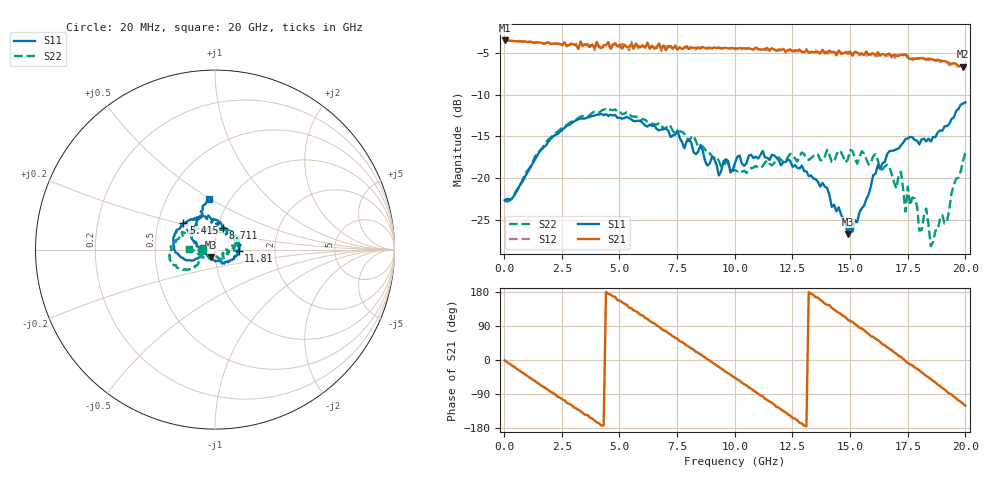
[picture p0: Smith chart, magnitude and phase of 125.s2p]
!Agilent Technologies,N5230A,US43500223,A.07.50.48
!Agilent N5230A: A.07.50.48
!Date: Tuesday, September 15, 2015 20:15:57
!Correction: S11(Full 2 Port(1,2))
!S21(Full 2 Port(1,2))
!S12(Full 2 Port(1,2))
!S22(Full 2 Port(1,2))
!S2P File: Measurements: S11, S21, S12, S22:
# Hz S  RI  R 50
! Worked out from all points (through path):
!   201 points, 20 MHz to 20 GHz, reference 50 ohm
!   highest |S21| = -3.50 dB at 20 MHz (marker M1); lowest = -6.6 dB at 19.9 GHz (marker M2)
!   group delay of S21, straight-line fit = 116 ps
!   lowest |S11| = -26.7 dB at 14.91 GHz (marker M3), VSWR 1.10, Z = 47.8 - j3.93 ohm
!   |S11| at or under -10 dB: start of sweep to end of sweep
!   |S22| runs from -28.2 to -11.7 dB; largest |S21 - S12| = 0.048
!   S11 on the Smith chart (normalised r, x): 20 MHz: 0.86, +0.00; 5.415 GHz: 0.67, +0.21; 8.711 GHz: 1.06, +0.26; 11.81 GHz: 1.31, -0.02; 20 GHz: 0.80, +0.49
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2e7  -0.0736 0.000765  0.668 -0.0104  0.668 -0.0107  -0.073 -0.000204
1.9181e9  -0.1538 -0.0604  0.119 -0.6413  0.1163 -0.6372  -0.1336 -0.1056
3.4166e9  -0.2271 0.0105  -0.4797 -0.3981  -0.4777 -0.3725  -0.214 -0.0977
4.5155e9  -0.2157 0.0958  -0.648 0.0598  -0.6482 0.0751  -0.2499 -0.0403
5.4146e9  -0.1758 0.147  -0.4542 0.4088  -0.45 0.3706  -0.2454 0.0158
6.7133e9  -0.0794 0.1765  0.0244 0.6407  0.0347 0.6339  -0.197 0.0809
8.7113e9  0.0435 0.119  0.5966 0.0685  0.5909 0.0716  -0.0951 0.1145
1.001e10  0.0965 0.0764  0.4062 -0.4366  0.4083 -0.4386  -0.0208 0.1096
1.09091e10  0.1286 0.0391  0.0611 -0.6037  0.0534 -0.6015  0.0396 0.1113
1.18082e10  0.1324 -0.00645  -0.3223 -0.4846  -0.3128 -0.485  0.0662 0.1141
1.34066e10  0.0764 -0.0637  -0.5645 0.0809  -0.5718 0.066  0.1145 0.0724
1.49051e10  -0.0214 -0.0411  -0.1537 0.5347  -0.1665 0.5456  0.1107 0.0675
1.57043e10  -0.0743 0.00833  0.1622 0.5507  0.1788 0.51  0.1219 0.0455
1.67033e10  -0.1307 0.0624  0.4852 0.2754  0.4817 0.2645  0.1144 0.0234
1.72028e10  -0.1335 0.0822  0.5439 0.0812  0.5306 0.0567  0.1091 -0.00405
1.74026e10  -0.1441 0.0927  0.551 -0.0243  0.5522 -0.0253  0.063 0.00106
1.78022e10  -0.1339 0.1031  0.4865 -0.1762  0.4964 -0.1601  0.0677 -0.0336
1.8002e10  -0.1259 0.0973  0.4639 -0.2408  0.4575 -0.243  0.0403 -0.027
1.83017e10  -0.1085 0.1254  0.3838 -0.3455  0.3745 -0.3433  0.0393 -0.0526
1.85015e10  -0.102 0.1308  0.3267 -0.3997  0.3257 -0.4018  0.0094 -0.0379
1.99001e10  -0.0437 0.2761  -0.194 -0.423  -0.2008 -0.4226  -0.1271 -0.00135
2e10  -0.0323 0.2822  -0.2378 -0.4016  -0.2379 -0.3927  -0.1421 0.00276
